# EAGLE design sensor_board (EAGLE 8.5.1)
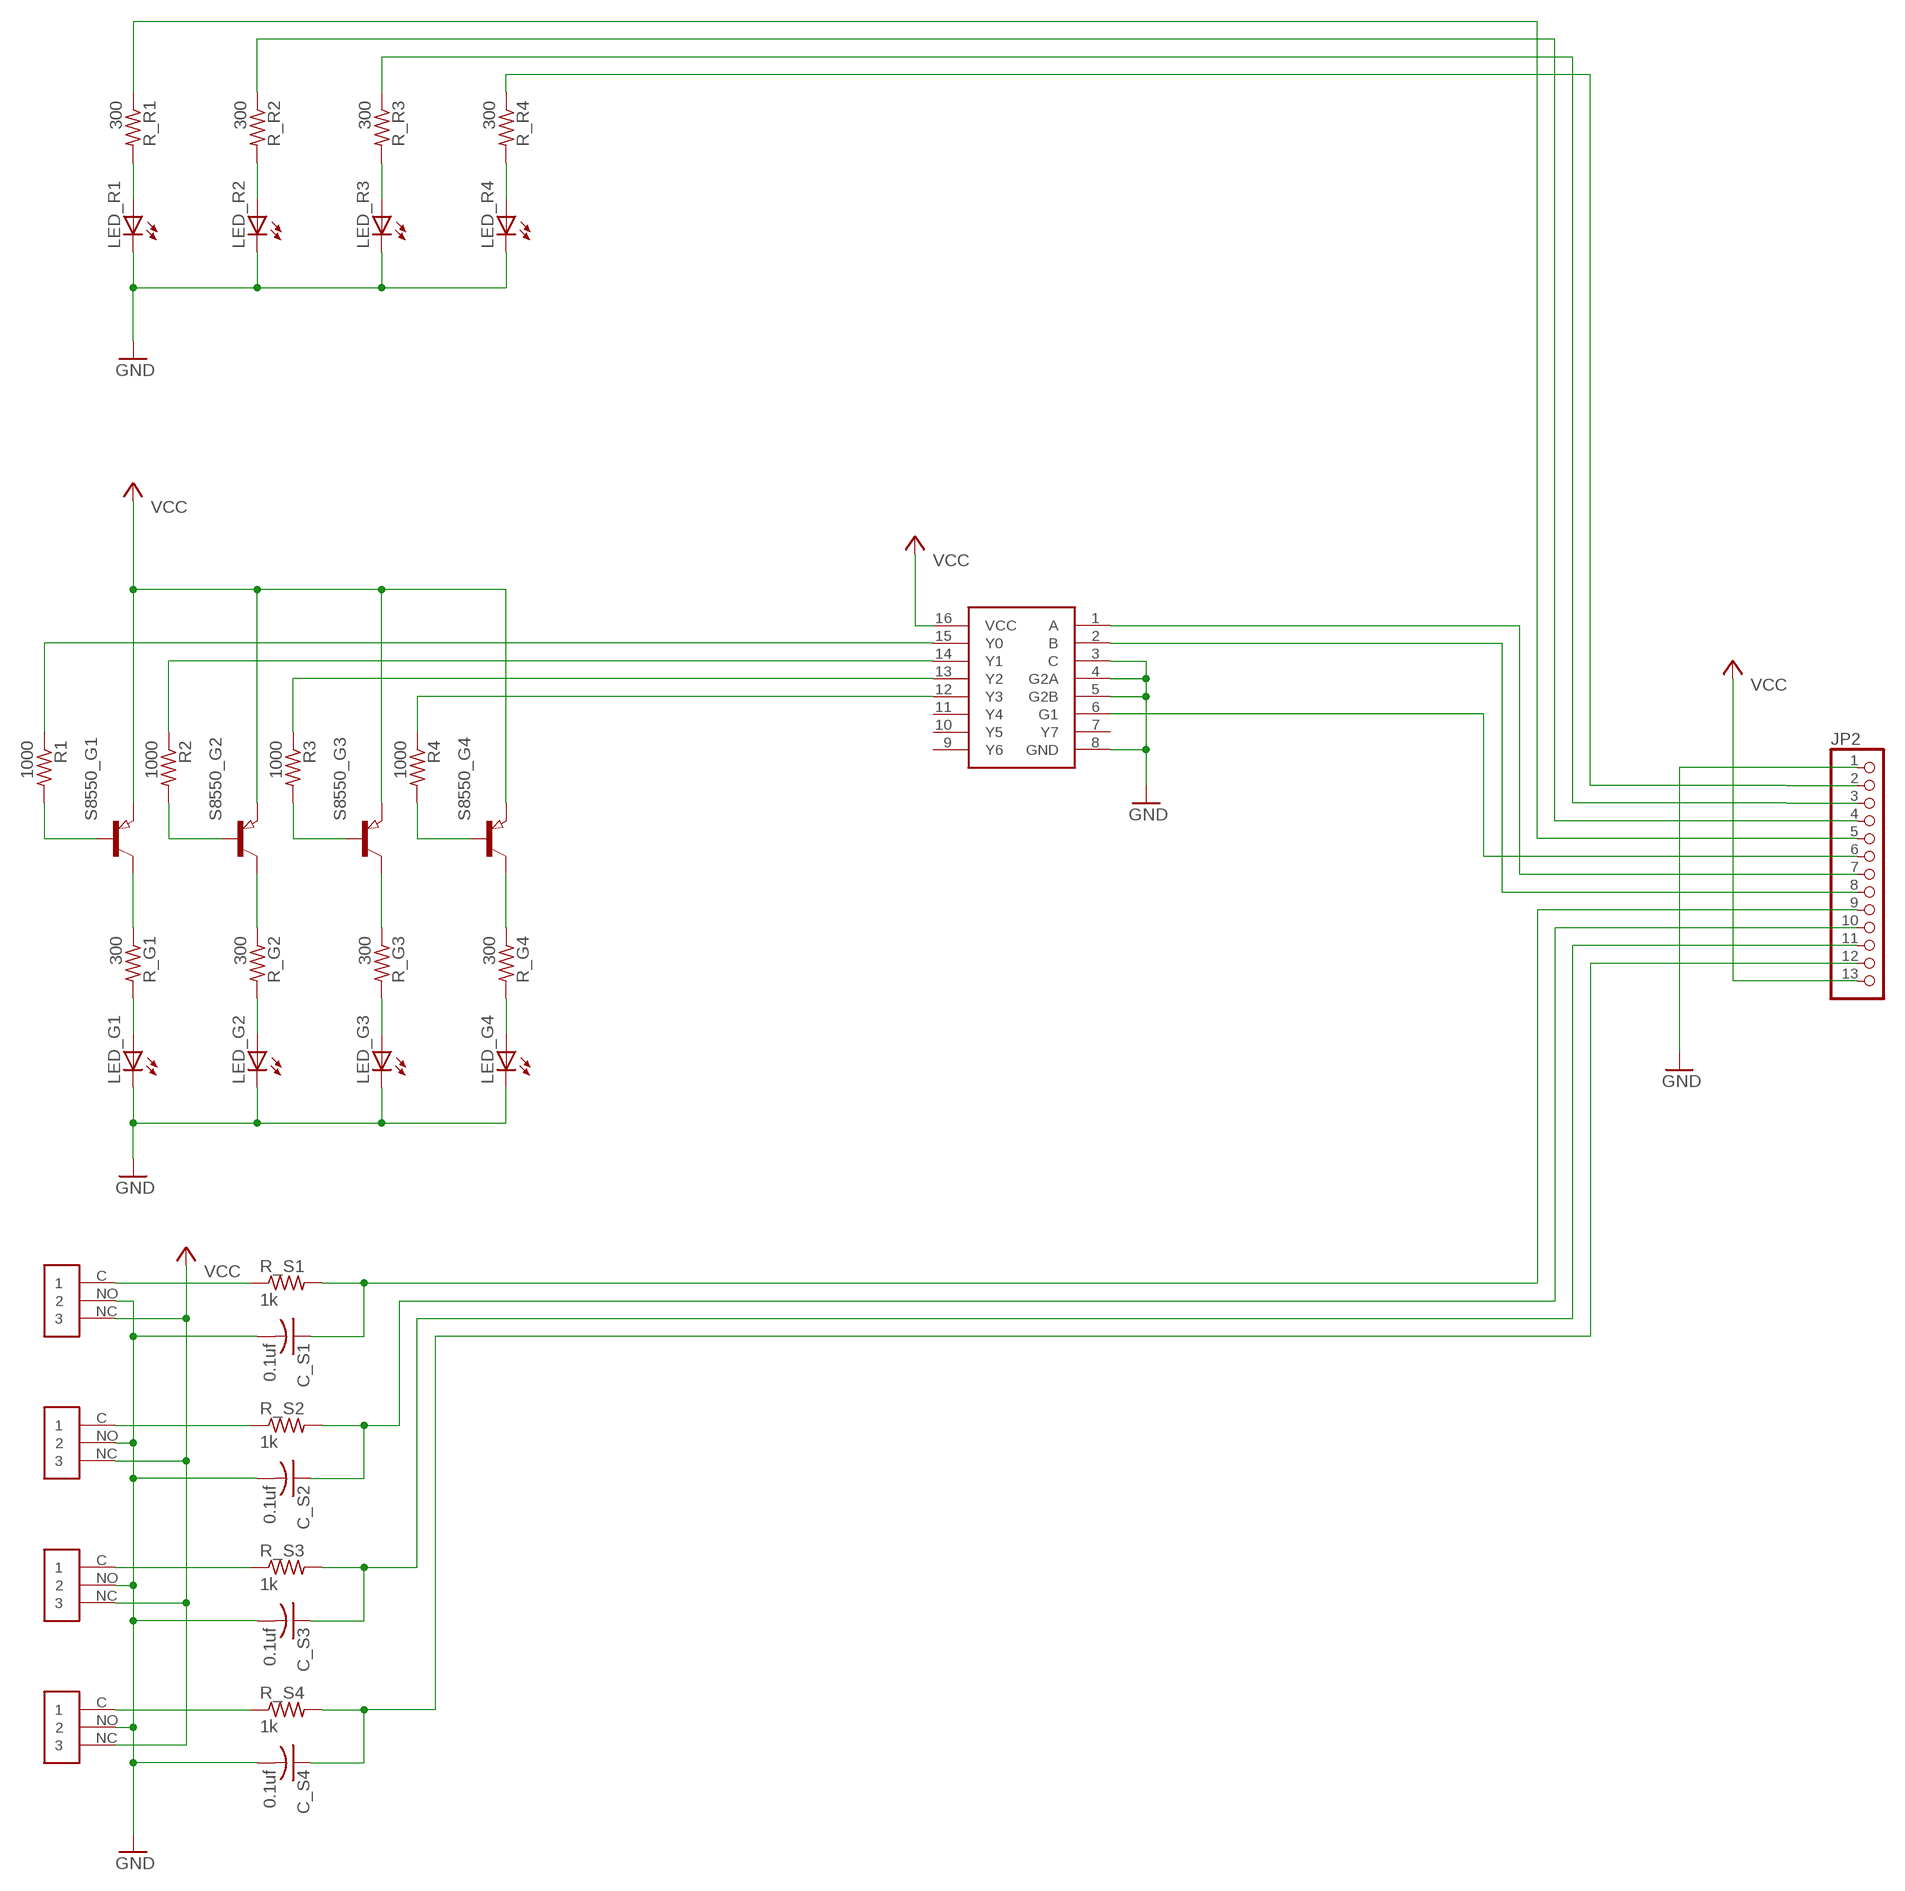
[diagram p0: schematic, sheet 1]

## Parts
C_S1  0.1uf  C-USC0805  [C0805]
C_S2  0.1uf  C-USC0805  [C0805]
C_S3  0.1uf  C-USC0805  [C0805]
C_S4  0.1uf  C-USC0805  [C0805]
DECODER  SN74LVC138A  [SO16]
JP2  PINHD-1X13  [1X13]
LED_G1  LEDSML0805  [SML0805]
LED_G2  LEDSML0805  [SML0805]
LED_G3  LEDSML0805  [SML0805]
LED_G4  LEDSML0805  [SML0805]
LED_R1  LEDSML0805  [SML0805]
LED_R2  LEDSML0805  [SML0805]
LED_R3  LEDSML0805  [SML0805]
LED_R4  LEDSML0805  [SML0805]
R1  1000  R-US_M0805  [M0805]
R2  1000  R-US_M0805  [M0805]
R3  1000  R-US_M0805  [M0805]
R4  1000  R-US_M0805  [M0805]
R_G1  300  R-US_M0805  [M0805]
R_G2  300  R-US_M0805  [M0805]
R_G3  300  R-US_M0805  [M0805]
R_G4  300  R-US_M0805  [M0805]
R_R1  300  R-US_M0805  [M0805]
R_R2  300  R-US_M0805  [M0805]
R_R3  300  R-US_M0805  [M0805]
R_R4  300  R-US_M0805  [M0805]
R_S1  1k  R-US_M0805  [M0805]
R_S2  1k  R-US_M0805  [M0805]
R_S3  1k  R-US_M0805  [M0805]
R_S4  1k  R-US_M0805  [M0805]
S8550_G1  PNP-TRANSISTOR_SOT23  [SOT23]
S8550_G2  PNP-TRANSISTOR_SOT23  [SOT23]
S8550_G3  PNP-TRANSISTOR_SOT23  [SOT23]
S8550_G4  PNP-TRANSISTOR_SOT23  [SOT23]
SW1  KW-10/A  [KW-10/A]
SW2  KW-10/A  [KW-10/A]
SW3  KW-10/A  [KW-10/A]
SW4  KW-10/A  [KW-10/A]

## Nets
GND: C_S1.2 C_S2.2 C_S3.2 C_S4.2 DECODER.3(C) DECODER.4(G2A) DECODER.5(G2B) DECODER.8(GND) JP2.1 LED_G1.C LED_G2.C LED_G3.C LED_G4.C LED_R1.C LED_R2.C LED_R3.C LED_R4.C SW1.NO SW2.NO SW3.NO SW4.NO
N$1: R_S2.1 SW2.C
N$2: DECODER.6(G1) JP2.6
N$3: R_S3.1 SW3.C
N$4: DECODER.1(A) JP2.7
N$5: LED_R4.A R_R4.2
N$6: LED_R3.A R_R3.2
N$7: LED_R2.A R_R2.2
N$8: LED_R1.A R_R1.2
N$9: C_S3.1 JP2.11 R_S3.2
N$10: DECODER.2(B) JP2.8
N$11: R_S1.1 SW1.C
N$12: R_S4.1 SW4.C
N$14: C_S4.1 JP2.12 R_S4.2
N$16: R_G1.1 S8550_G1.3(C)
N$17: LED_G1.A R_G1.2
N$18: DECODER.15(Y0) R1.1
N$19: DECODER.14(Y1) R2.1
N$20: DECODER.13(Y2) R3.1
N$21: DECODER.12(Y3) R4.1
N$23: C_S2.1 JP2.10 R_S2.2
N$24: R1.2 S8550_G1.1(B)
N$25: R_G2.1 S8550_G2.3(C)
N$26: LED_G2.A R_G2.2
N$27: R2.2 S8550_G2.1(B)
N$28: R_G3.1 S8550_G3.3(C)
N$29: LED_G3.A R_G3.2
N$30: R3.2 S8550_G3.1(B)
N$31: R_G4.1 S8550_G4.3(C)
N$32: LED_G4.A R_G4.2
N$33: R4.2 S8550_G4.1(B)
N$34: C_S1.1 JP2.9 R_S1.2
N$35: JP2.2 R_R4.1
N$37: JP2.3 R_R3.1
N$42: JP2.4 R_R2.1
N$43: JP2.5 R_R1.1
VCC: DECODER.16(VCC) JP2.13 S8550_G1.2(E) S8550_G2.2(E) S8550_G3.2(E) S8550_G4.2(E) SW1.NC SW2.NC SW3.NC SW4.NC
Unconnected: DECODER.7(Y7) DECODER.9(Y6) DECODER.10(Y5) DECODER.11(Y4)

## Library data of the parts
C_S1-C_S4 = adafruit:C-US: CAPACITOR, American symbol
DECODER = custom_package:SN74LVC138A
JP2 = adafruit:PINHD-1X13: PIN HEADER
LED_G1-LED_G4 LED_R1-LED_R4 = led:LED: LED
R1-R4 R_G1-R_G4 R_R1-R_R4 R_S1-R_S4 = adafruit:R-US_: RESISTOR, American symbol
S8550_G1-S8550_G4 = semicon-smd-ipc:PNP-TRANSISTOR_: PNP TRANSISTOR
SW1-SW4 = custom_package:KW-10/A

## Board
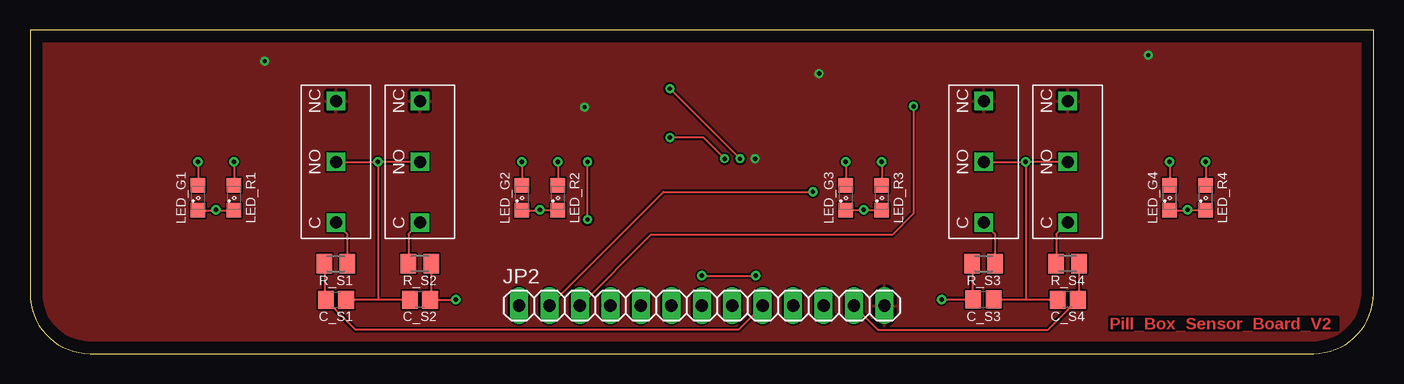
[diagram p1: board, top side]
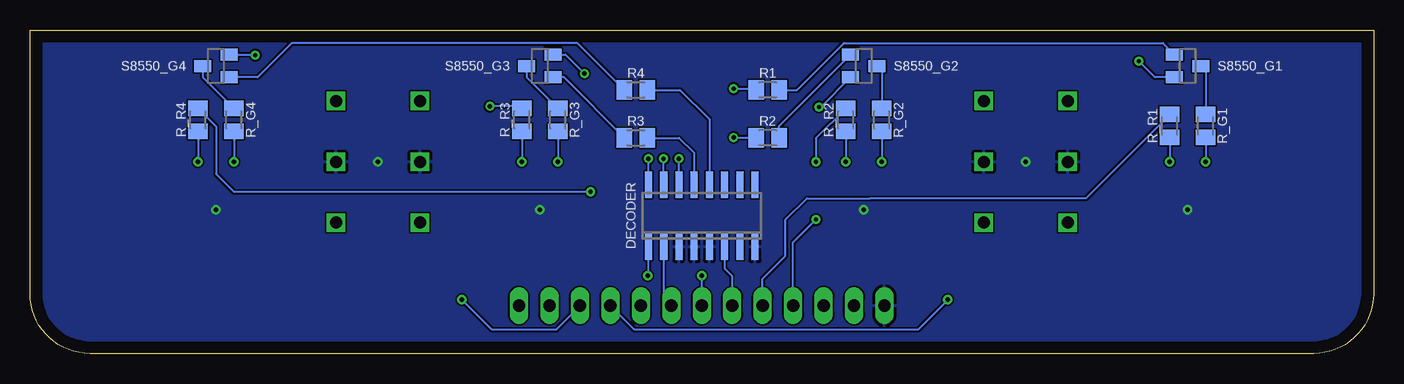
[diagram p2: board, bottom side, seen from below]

Size 112 x 27 mm. Coordinates in mm from the lower left corner, seen from the top.
Outline: 0,27 0,5 arc90 5,0 107,0 arc90 112,5 112,27 0,27
Copper layers (1*16): Top 0.035mm / dielectric 1.5mm / Bottom 0.035mm
Design rules "default": minimum track width 6mil, minimum drill 0.35mm, track to track 6mil, track to pad 6mil, pad to pad 6mil, via to via 6mil, smd to smd 6mil, copper to edge 40mil, drill to drill 6mil, minimum pad ring 10mil, minimum via ring 8mil, stop-mask expansion 4mil, vias tented up to drill 0mil, thermal gap 10mil

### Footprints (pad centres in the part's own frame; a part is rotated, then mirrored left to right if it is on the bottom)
C0805 = smd 1.3 x 1.5: 1 -0.85,0; 2 0.85,0
SO16 = smd 0.6 x 2.2: 1 -4.445,-2.6; 2 -3.175,-2.6; 3 -1.905,-2.6; 4 -0.635,-2.6; 5 0.635,-2.6; 6 1.905,-2.6; 7 3.175,-2.6; 8 4.445,-2.6; 9 4.445,2.6; 10 3.175,2.6; 11 1.905,2.6; 12 0.635,2.6; 13 -0.635,2.6; 14 -1.905,2.6; 15 -3.175,2.6; 16 -4.445,2.6
1X13 = drill 1.016 long: 1 -15.24,0; 2 -12.7,0; 3 -10.16,0; 4 -7.62,0; 5 -5.08,0; 6 -2.54,0; 7 0,0; 8 2.54,0; 9 5.08,0; 10 7.62,0; 11 10.16,0; 12 12.7,0; 13 15.24,0
SML0805 = smd 1.2 x 1.2: A 1.05,0; C -1.05,0
M0805 = smd 1.3 x 1.6: 1 -0.95,0; 2 0.95,0
SOT23 = smd 1 x 1.4: 1 -0.95,-1.1; 2 0.95,-1.1; 3 0,1.1
KW-10/A = drill 1 square: C -5.08,0; NC 5.08,0; NO 0,0

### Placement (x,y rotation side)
C_S1  25.5,4.5 0 top
C_S2  32.5,4.5 180 top
C_S3  79.49,4.52 0 top
C_S4  86.5,4.5 180 top
DECODER  56,11.5 0 bottom
JP2  56,4 0 top
LED_G1  14,13 90 top
LED_G2  41,13 90 top
LED_G3  68,13 90 top
LED_G4  95,13 90 top
LED_R1  17,13 90 top
LED_R2  44,13 90 top
LED_R3  71,13 90 top
LED_R4  98,13 90 top
R1  50.5,22 0 bottom
R2  50.5,18 0 bottom
R3  61.5,18 180 bottom
R4  61.5,22 180 bottom
R_G1  14,19 270 bottom
R_G2  41,19.5 270 bottom
R_G3  68,19.5 270 bottom
R_G4  95,19.5 270 bottom
R_R1  17,19 270 bottom
R_R2  44,19.5 270 bottom
R_R3  71,19.5 270 bottom
R_R4  98,19.5 270 bottom
R_S1  25.5,7.5 180 top
R_S2  32.5,7.5 0 top
R_S3  79.5,7.5 180 top
R_S4  86.5,7.5 0 top
S8550_G1  15.5,24 270 bottom
S8550_G2  42.5,24 270 bottom
S8550_G3  69.5,24 90 bottom
S8550_G4  96.5,24 90 bottom
SW1  25.5,16 90 top
SW2  32.5,16 90 top
SW3  79.5,16 90 top
SW4  86.5,16 90 top

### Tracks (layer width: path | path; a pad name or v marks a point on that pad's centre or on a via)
GND  (via drill 0.35)
  Top 0.152: SW1.NO v29,16 | SW2.NO v29,16 | v29,16 29,4.5 | 29,4.5 C_S1.2 | C_S2.2 29,4.5 | SW3.NO v83,16 | SW4.NO v83,16 | C_S4.2 83,4.5 | 83,4.5 80.36,4.5 C_S3.2 | v83,16 83,4.5 | LED_G4.C 96.45,11.95 | 96.45,11.95 v96.5,12 | LED_R4.C 96.45,11.95 | LED_G3.C 68.05,12 v69.5,12 69.55,11.95 LED_R3.C | LED_G1.C 15.45,11.95 v15.5,12 15.55,11.95 LED_R1.C 16.95,12 | LED_G2.C 42.45,11.95 | 42.45,11.95 v42.5,12 | LED_R2.C 42.45,11.95
  pour Bottom: 112.52,27.69 112.52,-0.25 113.03,-0.76 -1.52,-0.76 -1.52,27.18 -1.02,27.69
N$1
  Top 0.152: SW2.C 31.55,9.97 R_S2.1
N$2
  Bottom 0.152: DECODER.6 54.09,7.09 53.46,6.46 JP2.6
N$3
  Top 0.152: SW3.C 80.45,9.97 R_S3.1
N$4  (via drill 0.35)
  Top 0.152: v56,6.5 v60.5,6.5
  Bottom 0.152: JP2.7 v56,6.5 | v60.5,6.5 60.45,6.55 DECODER.1
N$5  (via drill 0.35)
  Top 0.152: v98,16 LED_R4.A
  Bottom 0.152: R_R4.2 v98,16
N$6  (via drill 0.35)
  Top 0.152: v71,16 LED_R3.A
  Bottom 0.152: R_R3.2 v71,16
N$7  (via drill 0.35)
  Top 0.152: v44,16 LED_R2.A
  Bottom 0.152: R_R2.2 v44,16
N$8  (via drill 0.35)
  Top 0.152: v17,16 LED_R1.A
  Bottom 0.152: R_R1.2 v17,16
N$9  (via drill 0.35)
  Top 0.152: R_S3.2 78.55,4.61 C_S3.1 76.02,4.52 v76,4.5
  Bottom 0.152: JP2.11 68.16,2 73.5,2 v76,4.5
N$10
  Bottom 0.152: DECODER.2 59.17,4.63 JP2.8
N$11
  Top 0.152: SW1.C 26.45,9.97 R_S1.1
N$12
  Top 0.152: SW4.C 85.55,9.97 R_S4.1
N$14
  Top 0.152: R_S4.2 87.45,4.6 C_S4.1 86.53,3.68 86.53,3.65 84.87,2 70.7,2 JP2.12
N$16
  Bottom 0.152: S8550_G1.3 14,23.6 R_G1.1
N$17  (via drill 0.35)
  Top 0.152: v14,16 LED_G1.A
  Bottom 0.152: R_G1.2 v14,16
N$18  (via drill 0.35)
  Top 0.152: v59.18,16.26 v53.34,22.1
  Bottom 0.152: DECODER.15 59.17,16.25 v59.18,16.26 | v53.34,22.1 51.55,22.1 R1.1
N$19  (via drill 0.35)
  Top 0.152: v57.91,16.26 56.13,18.03 v53.34,18.03
  Bottom 0.152: DECODER.14 57.91,16.25 v57.91,16.26 | v53.34,18.03 51.48,18.03 R2.1
N$20
  Bottom 0.152: R3.1 57.88,18 56.64,16.76 56.64,14.11 DECODER.13
N$21
  Bottom 0.152: R4.1 57.81,22 55.37,19.56 DECODER.12
N$23  (via drill 0.35)
  Top 0.152: R_S2.2 33.45,4.6 | 33.45,4.6 C_S2.1 | 33.45,4.6 33.55,4.5 v35.5,4.5
  Bottom 0.152: v35.5,4.5 38,2 61.62,2 JP2.10
N$24
  Bottom 0.152: R1.2 48.07,22 44.16,25.91 17.56,25.91 S8550_G1.1
N$25
  Bottom 0.152: S8550_G2.3 41,23.6 R_G2.1
N$26  (via drill 0.35)
  Top 0.152: v41,16 LED_G2.A
  Bottom 0.152: R_G2.2 v41,16
N$27
  Bottom 0.152: R2.2 49.55,19 S8550_G2.1
N$28
  Bottom 0.152: S8550_G3.3 70.6,23.05 R_G3.1
N$29  (via drill 0.35)
  Top 0.152: v68,16 LED_G3.A
  Bottom 0.152: R_G3.2 v68,16
N$30
  Bottom 0.152: R3.2 67.5,23.05 S8550_G3.1
N$31
  Bottom 0.152: S8550_G4.3 97.6,23.05 R_G4.1
N$32  (via drill 0.35)
  Top 0.152: v95,16 LED_G4.A
  Bottom 0.152: R_G4.2 v95,16
N$33
  Bottom 0.152: R4.2 66.36,25.91 90.17,25.91 93.03,23.05 S8550_G4.1
N$34
  Top 0.152: R_S1.2 24.55,4.6 C_S1.1 25.47,3.68 25.47,3.65 27.13,2 59.08,2 JP2.9
N$35  (via drill 0.35)
  Top 0.152: JP2.2 52.8,13.5 v65.28,13.5
  Bottom 0.152: R_R4.1 96.5,18.95 96.5,15 95,13.5 v65.28,13.5 65,13.5
N$37  (via drill 0.35)
  Top 0.152: v73.66,20.63 73.66,11.68 71.88,9.91 51.75,9.91 JP2.3
  Bottom 0.152: R_R3.1 71.18,20.63 v73.66,20.63
N$42  (via drill 0.35)
  Top 0.152: v46.48,11.18 v46.48,16
  Bottom 0.152: R_R2.1 46.48,17.97 v46.48,16 | JP2.4 48.38,9.28 v46.48,11.18
N$43
  Bottom 0.152: R_R1.1 24,12.95 41.4,12.95 41.97,12.95 47.24,12.95 49.02,11.18 49.02,8.13 50.92,6.23 JP2.5
VCC  (via drill 0.35)
  Bottom 0.152: 68.6,25.15 S8550_G3.2 67.37,24.95 v65.79,23.37 | S8550_G4.2 93.28,24.95 v93.22,24.89 | S8550_G2.2 46.08,20.57 v46.23,20.57 | S8550_G1.2 18.22,23.05 v19.56,24.38 | DECODER.16 60.45,16.25 v60.45,16.26
  pour Top: 112.52,26.92 112.52,-0.51 112.27,-0.76 -0.76,-0.76 -1.27,-0.25 -1.27,27.18 -0.76,27.69 111.76,27.69

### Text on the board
Top: Pill_Box_Sensor_Board_V2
